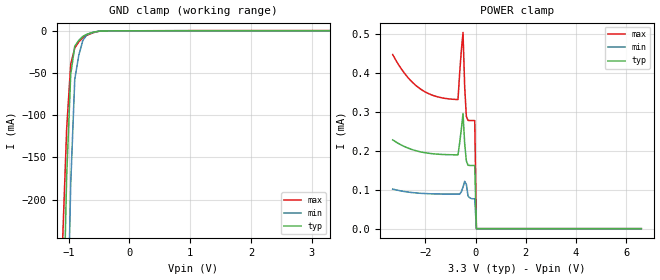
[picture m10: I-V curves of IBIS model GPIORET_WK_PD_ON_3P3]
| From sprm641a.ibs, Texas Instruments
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|RET_8MA_OPEN_DRAIN_3P3; 8MA_OPEN_DRAIN
|   Model Cell GPIORET_WK_PD_ON_3P3
|GPIORET_WK_PD_ON_3P3
[Model]   GPIORET_WK_PD_ON_3P3
Model_type   Input
Polarity   Non-Inverting
Vinl =  0.8
Vinh =  2
C_comp   5.345208p   4.561426p   6.022817p
[Model Spec]
Vinl   0.8   0.8   0.8
Vinh   2   2   2
[Temperature Range]   25   155   -40
[Voltage Range]   3.3   2.97   3.63
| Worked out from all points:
|   GND clamp passes 1 mA (typ) near -0.55 V on its own axis
| Nom Voltages:
|   BIASFET=3.3, VDD=1.2, VDDS=3.3, VSS=0
| Min Voltages:
|   BIASFET=2.97, VDD=1.08, VDDS=2.97, VSS=0
| Max Voltages:
|   BIASFET=3.63, VDD=1.32, VDDS=3.63, VSS=0
[POWER_clamp]
|   voltage   I(typ)   I(min)   I(max)
-3.3V     228.1uA    101.6uA    447.3uA
-2.767V   209.1uA    94.76uA    393.9uA
-2.167V   197uA      90.77uA    357.6uA
-700mV    189.6uA    88.78uA    331.6uA
-566.7mV  256.1uA    94.78uA    457.6uA
-500mV    295.6uA    106.8uA    504.2uA
-433.3mV  218.1uA    121.6uA    363.2uA
-366.7mV  173.9uA    113.9uA    287.8uA
-300mV    162.9uA    83.62uA    278.1uA
-33.33mV  162.2uA    76.8uA     277.6uA
33.33mV   0A         0A         0A
6.6V      0A         0A         0A
[GND_clamp]
|   voltage   I(typ)   I(min)   I(max)
-3.3V     -16.36A    -15.08A    -17.18A
-1.1V     -382.1mA   -717.8mA   -250.1mA
-1.033V   -173.3mA   -402.2mA   -116.4mA
-966.7mV  -52.02mA   -182.1mA   -39.8mA
-900mV    -18.2mA    -57.43mA   -20.33mA
-833.3mV  -11.36mA   -28.89mA   -13.17mA
-766.7mV  -6.626mA   -11.28mA   -8.158mA
-700mV    -4.013mA   -4.598mA   -5.306mA
-500mV    -405.1uA   -515.9uA   -494.1uA
-366.7mV  -78.5uA    -83.36uA   -110.5uA
3.3V      162.1uA    90.59uA    277.3uA
